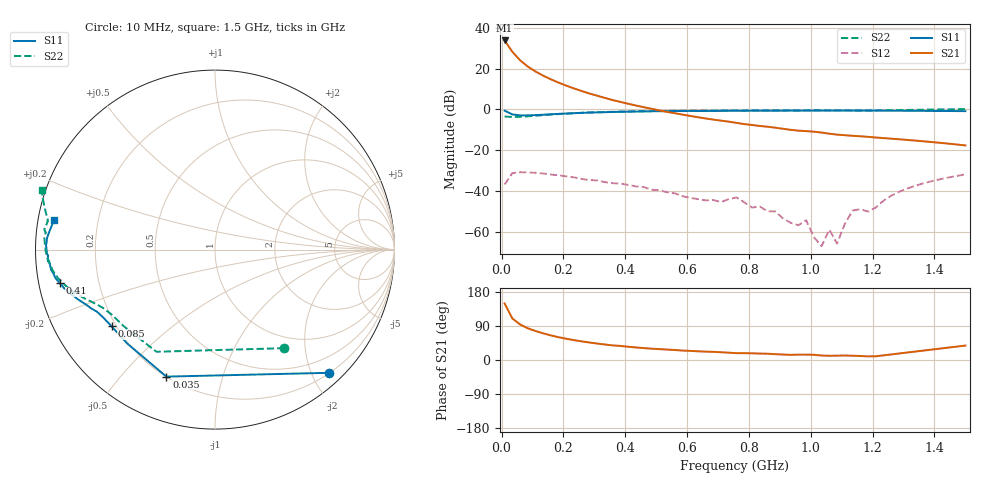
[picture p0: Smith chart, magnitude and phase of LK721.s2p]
! Date: Fri Jan 15 13:51:43 1999
!  POLYFET RF DEVICES
!  LK721 (EACH SIDE)
!  12.5Vdc		200ma
# MHZ  S  MA  R  50.0000
! SCATTERING PARAMETERS :
! Freq=MHz Mag[s11] Ang[s11] Mag[s21] Ang[s21] Mag[s12] Ang[s12] Mag[s22] Ang[s22]
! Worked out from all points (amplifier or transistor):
!   61 points, 10 MHz to 1.5 GHz, reference 50 ohm
!   highest |S21| = 33.8 dB at 10 MHz (marker M1)
!   |S21| within 3 dB of that: start of sweep to 23.53 MHz
!   unconditionally stable (mu >= 1): 555.5 MHz to 1.331 GHz; 1.338 GHz to 1.367 GHz
!   at 260 MHz: K = 0.28, MSG = 21.5 dB, |S12| = -34.1 dB
!   at 760 MHz: K = 1.46, MAG = 14.2 dB, |S12| = -43.1 dB
!   at 1.5 GHz: K = -1.07, MSG = 7.1 dB, |S12| = -31.8 dB
!   S11 on the Smith chart (normalised r, x): 10 MHz: 0.21, -2.26; 35 MHz: 0.20, -0.67; 85 MHz: 0.18, -0.32; 410 MHz: 0.06, -0.11; 1.5 GHz: 0.05, +0.09
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10  0.9334 -47.3  48.94 149.2  0.01457 59.5  0.6714 -54.9
35  0.7577 -110.9  25.85 109.7  0.02764 21.2  0.6561 -119.8
60  0.7162 -133.1  16 93.8  0.02916 4.3  0.663 -139.6
85  0.7172 -143.4  11.24 83.7  0.02869 -4.5  0.6801 -147.8
110  0.7287 -148.7  8.499 76.5  0.02815 -11.2  0.7027 -152.4
135  0.7423 -152.1  6.694 70.3  0.02706 -17.7  0.7281 -155.4
160  0.7638 -154.6  5.46 64.8  0.02552 -22.2  0.7521 -157.6
210  0.7967 -158.5  3.818 56.0  0.02297 -30.2  0.7911 -160.8
260  0.8264 -161.6  2.809 49.0  0.01979 -37.0  0.8299 -163.8
335  0.8581 -164.9  1.912 40.8  0.01659 -44.8  0.8646 -167.4
410  0.8834 -167.7  1.377 34.9  0.01419 -45.1  0.8953 -170.7
510  0.9058 -170.5  0.9489 28.7  0.01059 -54.4  0.9175 -174.1
760  0.9306 -176.0  0.4695 18.0  0.007 -47.9  0.9446 179.1
935  0.9396 -178.7  0.3172 13.6  0.00168 -24.2  0.9488 174.6
985  0.9375 -178.6  0.2954 14.2  0.00195 -4.9  0.9522 173.9
1010  0.9373 -179.3  0.2859 13.8  0.00075 26.5  0.9578 173.2
1035  0.9392 179.5  0.272 11.8  0.00045 9.6  0.9521 172.5
1060  0.9415 178.7  0.2553 11.1  0.00114 33.5  0.9515 171.8
1085  0.9433 178.2  0.2423 11.5  0.00052 65.0  0.9483 171.4
1135  0.9407 178.2  0.2268 11.3  0.00334 76.7  0.9453 170.5
1260  0.9338 175.1  0.1929 14.7  0.00772 -18.8  0.9607 168.1
1500  0.9102 169.6  0.1317 38.1  0.02572 -159.3  1.022 161.0
